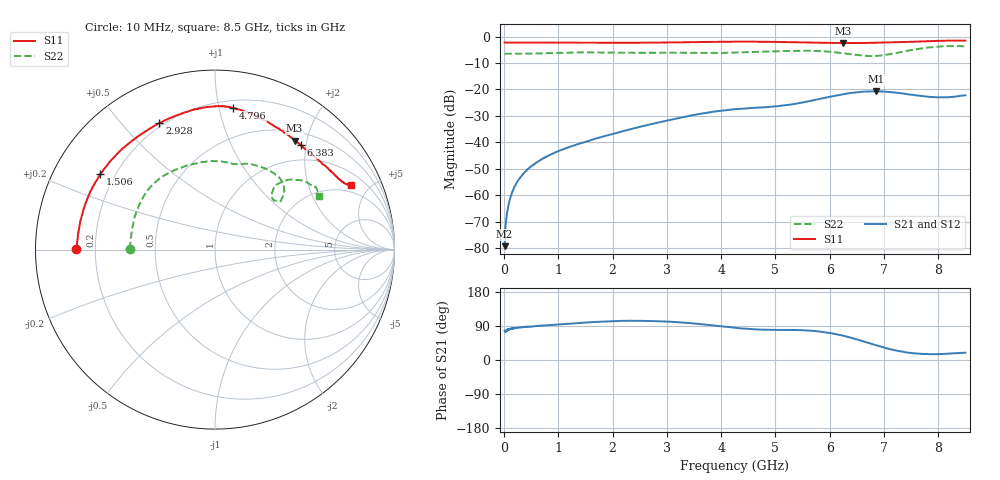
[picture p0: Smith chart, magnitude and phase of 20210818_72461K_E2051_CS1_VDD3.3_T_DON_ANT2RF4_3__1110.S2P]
!Agilent Technologies,E5071C,MY46417908,A.11.23
!Date: Wed Aug 18 14:33:38 2021
!Data & Calibration Information:
!Freq	S11:SOLT2(ON)	S21:SOLT2(ON)	S12:SOLT2(ON)	S22:SOLT2(ON)
!PortZ  Port1:50+j0  Port2:50+j0
!Above PortZ is port z conversion or system Z0 setting when saving the data.
!When reading, reference impedance value at option line is always used.
# Hz S dB R 50
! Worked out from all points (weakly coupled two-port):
!   1601 points, 10 MHz to 8.5 GHz, reference 50 ohm
!   highest |S21| = -20.72 dB at 6.86 GHz (marker M1); lowest = -79.3 dB at 10 MHz (marker M2)
!   lowest |S11| = -2.5 dB at 6.25 GHz (marker M3), VSWR 7.05, Z = 32.1 + j89.5 ohm
!   |S11| at or under -10 dB: nowhere
!   |S22| runs from -7.4 to -3.6 dB; largest |S21 - S12| = 0.00044
!   S11 on the Smith chart (normalised r, x): 10 MHz: 0.13, +0.00; 1.506 GHz: 0.15, +0.29; 2.928 GHz: 0.18, +0.64; 4.796 GHz: 0.26, +1.10; 6.383 GHz: 0.71, +1.90; 8.5 GHz: 1.56, +3.80
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1e7  -2.24 179.7  -79.27 77.3  -78.88 74.3  -6.47 179.5
6.836875e7  -2.27 178.4  -65.13 82.3  -65.08 80.7  -6.50 177.9
1.16125e8  -2.28 177.3  -60.93 82.1  -60.93 82.4  -6.50 176.4
2.063312e8  -2.30 175.2  -56.36 83.6  -56.23 83.6  -6.51 173.8
3.28375e8  -2.30 172.5  -52.52 86.7  -52.58 86.3  -6.49 170.4
4.716438e8  -2.30 169.3  -49.54 88.3  -49.55 88.4  -6.45 166.6
7.422625e8  -2.32 163.1  -45.90 91.0  -45.82 91.2  -6.32 158.2
1.426769e9  -2.33 148.5  -40.27 97.9  -40.30 97.9  -6.00 135.4
1.506362e9  -2.34 146.7  -39.76 98.9  -39.76 99.0  -6.00 132.8
2.063519e9  -2.35 134.4  -36.52 102.8  -36.50 102.8  -6.10 115.2
2.843538e9  -2.29 115.7  -32.52 102.2  -32.53 102.1  -6.15 95.4
2.928438e9  -2.28 113.8  -32.15 101.7  -32.16 101.6  -6.13 93.7
4.255e9  -1.96 89.8  -27.49 85.1  -27.48 85.0  -6.11 74.1
4.796238e9  -1.99 82.8  -26.77 79.9  -26.77 80.0  -5.72 66.4
5.671769e9  -2.28 67.4  -24.23 77.2  -24.25 77.3  -5.40 47.9
6.25015e9  -2.48 53.9  -21.82 64.1  -21.85 64.0  -6.34 38.3
6.382806e9  -2.46 50.6  -21.37 59.1  -21.39 59.0  -6.73 36.8
6.860369e9  -2.33 39.8  -20.72 38.7  -20.75 38.6  -7.32 42.6
7.088538e9  -2.21 35.7  -20.96 29.4  -20.98 29.2  -6.73 45.6
7.613856e9  -1.91 28.5  -22.31 17.1  -22.31 17.0  -4.74 42.4
8.086112e9  -1.60 25.8  -22.99 15.8  -22.97 15.7  -3.69 32.7
8.5e9  -1.53 25.6  -22.23 19.3  -22.24 19.0  -3.73 27.3
